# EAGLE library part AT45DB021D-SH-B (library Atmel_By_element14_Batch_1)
2-megabit DataFlash
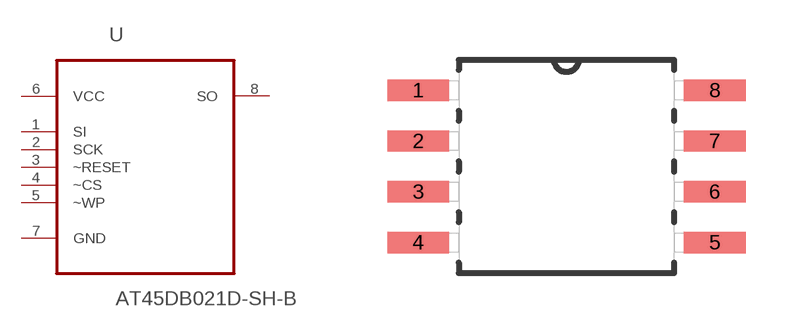
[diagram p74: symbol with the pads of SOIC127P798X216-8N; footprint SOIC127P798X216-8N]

Designator prefix U

## AT45DB021D-SH-B (MPN: AT45DB021D-SH-B; OC_FARNELL: 1715456; OC_NEWARK: 14R9984; PACKAGE: SOIC-8; SUPPLIER: Atmel)  [SOIC127P798X216-8N]
1  SI  in
2  SCK  in
3  ~RESET  in
4  ~CS  in
5  ~WP  in
6  VCC  pwr
7  GND  pas
8  SO  out

## Footprint SOIC127P798X216-8N (pad centres in mm)
smd 1.549 x 0.533: 1 -3.708,1.905; 2 -3.708,0.635; 3 -3.708,-0.635; 4 -3.708,-1.905; 5 3.708,-1.905; 6 3.708,-0.635; 7 3.708,0.635; 8 3.708,1.905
